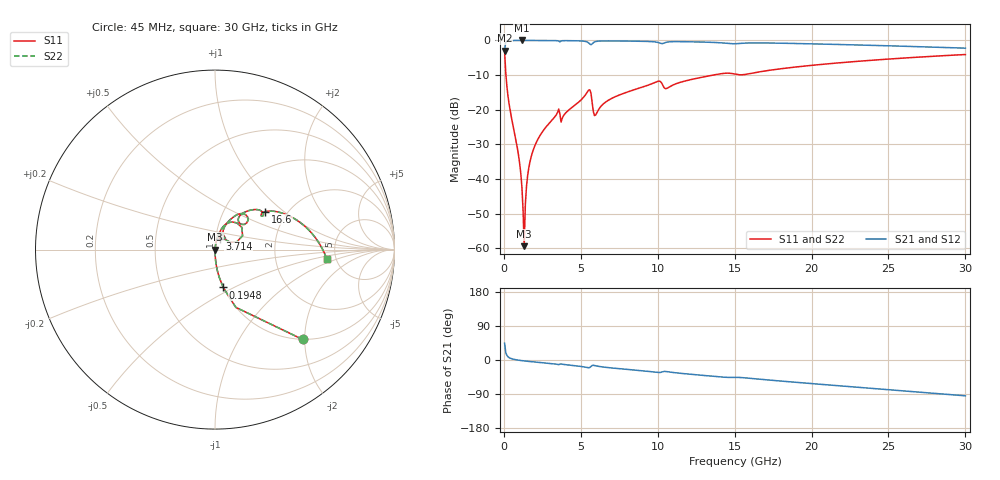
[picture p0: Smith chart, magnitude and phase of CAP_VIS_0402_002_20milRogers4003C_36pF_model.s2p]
! S-parameter model data by Modelithics Inc.  support@modelithics.com  813-866-6335  Tampa FL USA
! S-Parameter data specifications:
! Substrate: 20-mil Rogers 4003C, substrate thickness, H=0.508mm, Dielectric constant, Er=3.75
! PCB Mounting Pad Footprint: Pad width, PadW=0.50mm , Pad length, PadL=0.50mm , Pad gap, PadG (edge-to-edge)=0.40mm , Reference planes=1.4mm apart
! Created Wed Nov 18 12:54:29 2015
# hz S ma R 50
! 2 Port Network Data from SP1.SP block
! freq  magS11  angS11  magS21  angS21  magS12  angS12  magS22  angS22
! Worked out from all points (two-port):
!   401 points, 45 MHz to 30 GHz, reference 50 ohm
!   highest |S21| = -0.01 dB at 1.168 GHz (marker M1); lowest = -2.9 dB at 45 MHz (marker M2)
!   |S21| within 3 dB of the highest: start of sweep to end of sweep
!   lowest |S11| = -59.4 dB at 1.318 GHz (marker M3), VSWR 1.00, Z = 50.1 + j0.0414 ohm
!   |S11| at or under -10 dB: 132.7 MHz to 13.6 GHz (13.46 GHz wide, 196 % of centre)
!   |S22| runs from -59.4 to -3.1 dB; largest |S21 - S12| = 0
!   S11 on the Smith chart (normalised r, x): 45 MHz: 1.00, -1.95; 194.8 MHz: 1.00, -0.44; 3.714 GHz: 1.04, +0.13; 16.6 GHz: 1.56, +0.75; 30 GHz: 4.21, -0.76
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4.5e7  0.6989 -45.7  0.715 44.3  0.715 44.3  0.6989 -45.7
1.94775e8  0.2158 -77.8  0.976 12.1  0.976 12.1  0.2158 -77.8
4.194375e8  0.09381 -85.0  0.995 4.6  0.995 4.6  0.09381 -85.0
9.4365e8  0.02249 -88.3  0.9989 -0.4  0.9989 -0.4  0.02249 -88.3
1.168312e9  0.007765 -84.9  0.999 -1.7  0.999 -1.7  0.007765 -84.9
1.318088e9  0.001074 22.6  0.999 -2.4  0.999 -2.4  0.001074 22.6
1.467862e9  0.007831 79.4  0.9989 -3.1  0.9989 -3.1  0.007831 79.4
1.692525e9  0.01767 82.4  0.9987 -4.1  0.9987 -4.1  0.01767 82.4
1.992075e9  0.02953 82.4  0.9983 -5.3  0.9983 -5.3  0.02953 82.4
3.414938e9  0.0853 76.4  0.9925 -11.1  0.9925 -11.1  0.0853 76.4
3.714488e9  0.06624 67.4  0.9838 -10.4  0.9838 -10.4  0.06624 67.4
5.062462e9  0.1419 69.4  0.9815 -17.3  0.9815 -17.3  0.1419 69.4
5.511788e9  0.1926 50.3  0.9197 -20.4  0.9197 -20.4  0.1926 50.3
5.961112e9  0.08385 51.1  0.9632 -15.2  0.9632 -15.2  0.08385 51.1
7.084425e9  0.1486 66.7  0.9837 -21.3  0.9837 -21.3  0.1486 66.7
1.007992e10  0.2587 47.9  0.9254 -33.0  0.9254 -33.0  0.2587 47.9
1.060414e10  0.2037 49.7  0.9455 -30.7  0.9455 -30.7  0.2037 49.7
1.50225e10  0.3261 35.2  0.896 -46.0  0.896 -46.0  0.3261 35.2
1.659514e10  0.3514 37.1  0.9214 -50.6  0.9214 -50.6  0.3514 37.1
2.003996e10  0.4377 26.9  0.8925 -62.4  0.8925 -62.4  0.4377 26.9
2.505742e10  0.5394 10.9  0.8359 -78.6  0.8359 -78.6  0.5394 10.9
3e10  0.6261 -5.0  0.7733 -94.5  0.7733 -94.5  0.6261 -5.0
